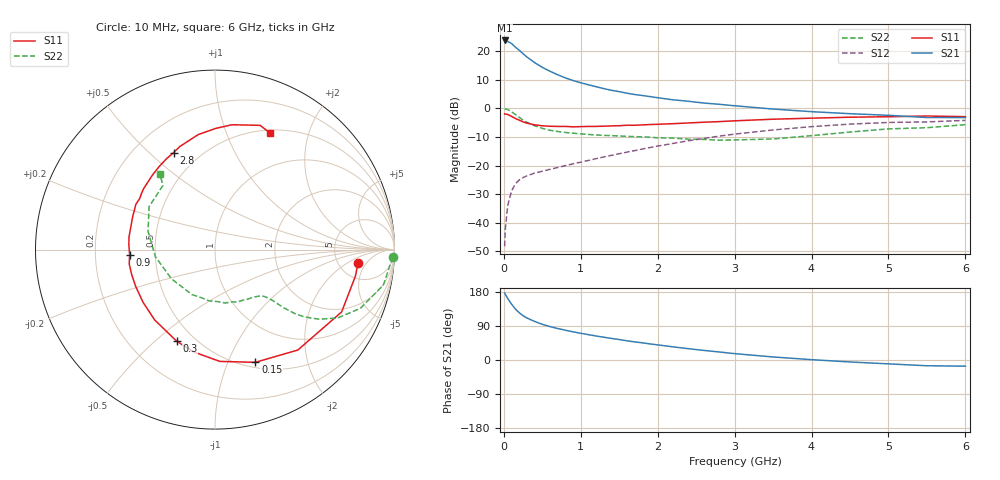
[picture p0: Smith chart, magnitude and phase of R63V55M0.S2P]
! SIEMENS Small Signal Semiconductors
! BFR193
! Si NPN RF Bipolar Junction Transistor in SOT23
! VCE = 3.5 V  IC = 5 mA
! Common Emitter S-Parameters:  May  1996
# GHz  S  MA  R  50
!  f  S11  S21  S12  S22
! GHz  MAG  ANG  MAG  ANG  MAG  ANG  MAG  ANG
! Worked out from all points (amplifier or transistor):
!   36 points, 10 MHz to 6 GHz, reference 50 ohm
!   highest |S21| = 23.8 dB at 10 MHz (marker M1)
!   |S21| within 3 dB of that: start of sweep to 180.4 MHz
!   unconditionally stable (mu >= 1): 897.8 MHz to 2.023 GHz
!   at 250 MHz: K = 0.43, MSG = 21.7 dB, |S12| = -24.2 dB
!   at 1.4 GHz: K = 1.06, MAG = 9.8 dB, |S12| = -16.4 dB
!   at 6 GHz: K = 0.96, MSG = 0.5 dB, |S12| = -4.2 dB
!   lowest NFmin = 1.20 dB at 450 MHz
!   S11 on the Smith chart (normalised r, x): 10 MHz: 7.61, -3.25; 150 MHz: 0.56, -1.26; 300 MHz: 0.40, -0.59; 900 MHz: 0.35, -0.03; 2.8 GHz: 0.36, +0.60; 6 GHz: 0.54, +1.44
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0.01  0.8004 -5.5  15.44 176.7  0.0039 86.2  0.9914 -2.4
0.02  0.7959 -10.8  15.16 172.8  0.008 85.2  0.9796 -4.9
0.05  0.7864 -26.2  14.84 162.6  0.0198 77.2  0.9588 -11.9
0.1  0.7253 -50.5  13.65 147.4  0.0359 67.0  0.8736 -22.0
0.15  0.6671 -70.3  11.81 134.5  0.0481 58.7  0.7826 -29.1
0.2  0.6236 -87.5  10.4 124.8  0.0563 53.5  0.6995 -33.7
0.25  0.5823 -101.8  9.043 116.8  0.0617 50.1  0.6249 -36.9
0.3  0.5532 -112.7  7.921 110.9  0.0663 48.6  0.5711 -38.7
0.4  0.5164 -130.6  6.332 101.8  0.074 46.7  0.4991 -40.3
0.5  0.4968 -143.8  5.224 94.2  0.0798 47.4  0.4477 -41.1
0.6  0.4873 -154.9  4.464 88.2  0.0861 49.1  0.4147 -41.8
0.7  0.4846 -163.2  3.88 83.1  0.0927 50.4  0.3948 -42.6
0.9  0.4764 -176.7  3.077 74.4  0.1077 53.1  0.3688 -44.6
1.1  0.4844 171.7  2.588 66.9  0.1232 56.0  0.3506 -48.1
1.3  0.4884 162.0  2.22 60.1  0.1416 57.8  0.3375 -52.0
1.6  0.508 150.2  1.844 50.7  0.172 59.0  0.3246 -59.5
2.2  0.5409 130.5  1.414 34.7  0.2445 57.3  0.3033 -79.0
2.8  0.5879 113.1  1.181 21.2  0.3275 51.0  0.2784 -106.5
3.5  0.6477 98.3  0.975 8.0  0.4202 40.5  0.2921 -146.2
4.5  0.7019 82.3  0.809 -5.2  0.5317 23.6  0.3865 164.8
5.5  0.7365 70.0  0.693 -15.2  0.5808 6.4  0.4603 129.1
6  0.7173 64.5  0.692 -16.3  0.6181 1.4  0.52 126.1
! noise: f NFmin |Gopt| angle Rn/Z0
0.45  1.2  0.26  102  0.14
0.9  1.25  0.38  145  0.12
1.8  2.05  0.56  -161  0.12
